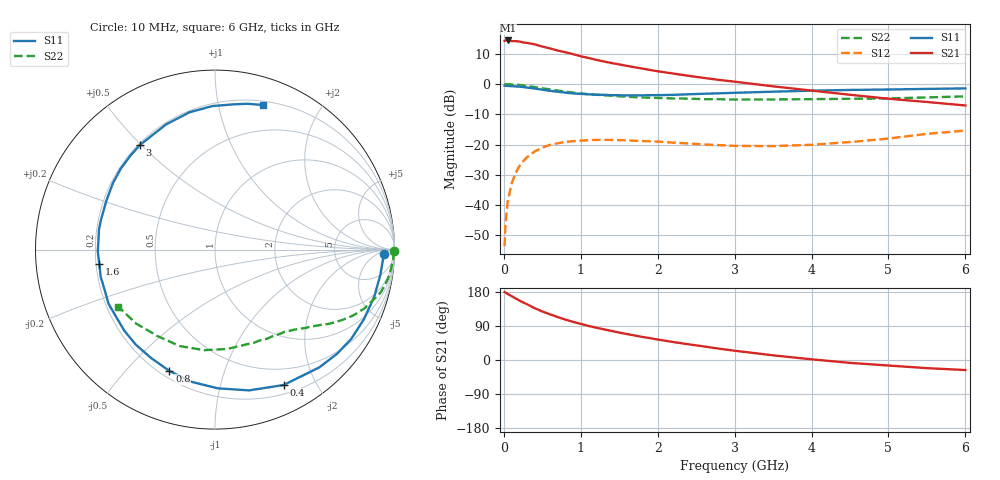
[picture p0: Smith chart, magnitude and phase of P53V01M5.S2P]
! SIEMENS Small Signal Semiconductors
! BFP183
! Si NPN RF Bipolar Junction Transistor in SOT143
! VCE = 3 V  IC = 1.5 mA
! Common Emitter S-Parameters:  March  1996
# GHz  S  MA  R  50
!  f  S11  S21  S12  S22
! GHz  MAG  ANG  MAG  ANG  MAG  ANG  MAG  ANG
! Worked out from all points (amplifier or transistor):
!   36 points, 10 MHz to 6 GHz, reference 50 ohm
!   highest |S21| = 14.4 dB at 50 MHz (marker M1)
!   |S21| within 3 dB of that: start of sweep to 652.6 MHz
!   unconditionally stable (mu >= 1): 2.263 GHz to end of sweep
!   at 250 MHz: K = 0.11, MSG = 19.7 dB, |S12| = -25.5 dB
!   at 1.4 GHz: K = 0.60, MSG = 12.7 dB, |S12| = -18.5 dB
!   at 6 GHz: K = 1.01, MAG = 3.5 dB, |S12| = -15.4 dB
!   S11 on the Smith chart (normalised r, x): 10 MHz: 27, -13; 400 MHz: 0.30, -1.59; 800 MHz: 0.24, -0.67; 1.6 GHz: 0.21, -0.06; 3 GHz: 0.21, +0.50; 6 GHz: 0.24, +1.36
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0.01  0.9418 -1.6  5.187 179.2  0.0021 90.6  0.9994 -0.6
0.02  0.9373 -3.4  5.231 178.3  0.0046 91.2  0.9955 -1.2
0.05  0.9322 -8.5  5.257 174.3  0.0114 88.5  0.994 -3.0
0.1  0.9254 -16.4  5.119 168.8  0.0225 79.3  0.9871 -6.1
0.15  0.916 -25.0  5.122 162.9  0.0333 75.1  0.9788 -9.1
0.2  0.9077 -33.2  5.056 157.3  0.0438 70.8  0.9669 -11.9
0.3  0.8766 -48.4  4.792 147.3  0.0618 62.5  0.9317 -16.9
0.4  0.8459 -63.1  4.54 136.9  0.077 54.5  0.8936 -21.6
0.5  0.807 -76.4  4.165 128.1  0.0891 47.1  0.8527 -25.5
0.6  0.7732 -88.8  3.882 120.5  0.099 41.3  0.8157 -28.5
0.8  0.7222 -110.6  3.355 106.6  0.1106 31.2  0.7516 -33.5
0.9  0.701 -120.6  3.119 100.7  0.114 27.2  0.7229 -35.5
1.1  0.6779 -138.1  2.702 89.9  0.1185 20.1  0.6813 -39.1
1.3  0.6654 -153.1  2.362 80.9  0.1198 14.6  0.6533 -42.3
1.6  0.6498 -173.1  2.001 68.5  0.1179 8.9  0.6206 -46.5
1.8  0.6516 175.2  1.803 60.9  0.1145 6.8  0.6 -49.7
2.2  0.6637 155.8  1.494 47.5  0.1079 3.5  0.5793 -56.3
3  0.7176 125.6  1.096 24.5  0.0952 5.9  0.5561 -71.9
3.5  0.7487 111.4  0.918 12.3  0.0945 11.8  0.5578 -82.9
4.5  0.7999 91.0  0.666 -7.6  0.1102 22.4  0.5723 -110.1
5.5  0.8325 77.5  0.506 -21.5  0.1504 25.1  0.6022 -136.8
6  0.8487 71.6  0.443 -26.5  0.1708 22.0  0.626 -149.5
